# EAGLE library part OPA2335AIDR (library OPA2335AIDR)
Dual 0.05uV/C max, single-supply CMOS operational amplifier Source: Datasheet
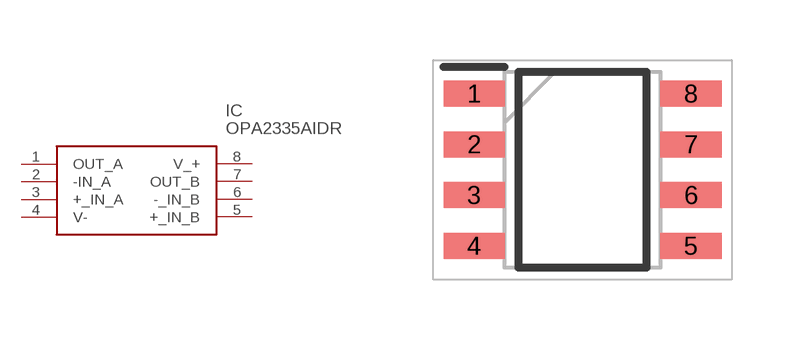
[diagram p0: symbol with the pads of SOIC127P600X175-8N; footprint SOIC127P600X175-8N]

Designator prefix IC

## OPA2335AIDR (Arrow_Part_Number: OPA2335AIDR; Arrow_Price-Stock: https://www.arrow.com/en/products/opa2335aidr/texas-instruments?region=nac; Description: Dual 0.05uV/C max, single-supply CMOS operational amplifier; Height: 1.75mm; Manufacturer_Name: Texas Instruments; Manufacturer_Part_Number: OPA2335AIDR; Mouser_Part_Number: 595-OPA2335AIDR; Mouser_Price-Stock: https://www.mouser.co.uk/ProductDetail/Texas-Instruments/OPA2335AIDR?qs=7nS3%252BbEUL6uJHBhnbuRjDw%3D%3D)  [SOIC127P600X175-8N]
1  OUT_A
2  -IN_A
3  +_IN_A
4  V-
5  +_IN_B
6  -_IN_B
7  OUT_B
8  V_+

## Footprint SOIC127P600X175-8N (pad centres in mm)
D0008A
smd 1.528 x 0.65: 1 -2.711,1.905; 2 -2.711,0.635; 3 -2.711,-0.635; 4 -2.711,-1.905; 5 2.711,-1.905; 6 2.711,-0.635; 7 2.711,0.635; 8 2.711,1.905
